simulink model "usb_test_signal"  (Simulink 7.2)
settings: Solver=ode45  StartTime=0.0  StopTime=10.0  RelTol=1e-3

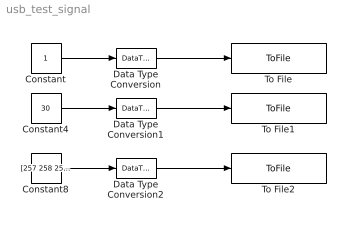
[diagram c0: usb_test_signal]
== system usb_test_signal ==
  Constant : Constant  OutDataTypeMode=uint16  OutDataType=sfix(16)  OutScaling=2^0  OutDataTypeStr=uint16  SampleTime=0.004
  Constant4 : Constant  Value=30  OutDataTypeMode=uint16  OutDataType=sfix(16)  OutScaling=2^0  OutDataTypeStr=uint16  SampleTime=0.004
  Constant8 : Constant  Value=[257 258 259 260 261 262 263 264 265 266 267 268 269 270 271 272 273 274 275 276 277 278 279 280 281 282 283 284 285 286]  OutDataTypeMode=uint16  OutDataType=sfix(16)  OutScaling=2^0  OutDataTypeStr=uint16  SampleTime=0.004
  Data Type Conversion : DataTypeConversion  OutDataType=sfix(16)  OutScaling=2^0
  Data Type Conversion1 : DataTypeConversion  OutDataType=sfix(16)  OutScaling=2^0
  Data Type Conversion2 : DataTypeConversion  OutDataType=sfix(16)  OutScaling=2^0
  To File : ToFile  Filename=usb_test_state.mat  MatrixName=usb_test_state
  To File1 : ToFile  Filename=usb_test_number.mat  MatrixName=usb_test_number
  To File2 : ToFile  Filename=usb_test_data.mat  MatrixName=usb_test_data
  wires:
  Data Type Conversion/1 -> To File/1
  Data Type Conversion1/1 -> To File1/1
  Data Type Conversion2/1 -> To File2/1
  Constant/1 -> Data Type Conversion/1
  Constant4/1 -> Data Type Conversion1/1
  Constant8/1 -> Data Type Conversion2/1
